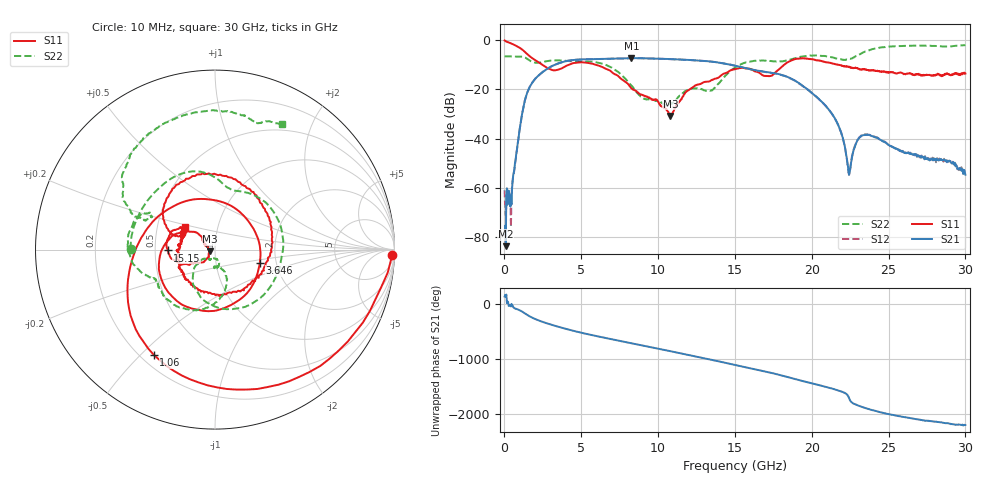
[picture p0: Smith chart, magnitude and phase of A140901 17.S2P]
!  2-Port S-parameters saved by WinCal
! VAR MeasName=S-Parameters (CALIBRATED_DATA) read from VNA (N5244A)
! VAR MeasDate=11/3/2014 9:28:11 AM
! VAR NAME=A140901 17
! VAR FILENAME=A140901 17.S2P
! VAR DATE=11/3/2014 9:28:11 AM
! VAR PHYS_PORTS=1,2
# Hz S RI R 50
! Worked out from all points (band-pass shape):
!   801 points, 10 MHz to 30 GHz, reference 50 ohm
!   highest |S21| = -7.29 dB at 8.257 GHz (marker M1); lowest = -83.7 dB at 84.97 MHz (marker M2)
!   |S21| within 3 dB of the highest: 3.168 GHz to 14.96 GHz (11.79 GHz wide, 130 % of centre)
!   lowest |S11| = -30.8 dB at 10.81 GHz (marker M3), VSWR 1.06, Z = 47.3 - j0.843 ohm
!   |S11| at or under -10 dB: 2.468 GHz to 4.195 GHz (1.727 GHz wide, 51.8 % of centre); 5.941 GHz to 18.2 GHz (12.26 GHz wide, 102 % of centre); 21.76 GHz to end of sweep
!   |S22| runs from -26.7 to -2.0 dB; largest |S21 - S12| = 0.005
!   S11 on the Smith chart (normalised r, x): 10 MHz: 21, -54; 1.06 GHz: 0.25, -0.55; 3.646 GHz: 1.64, -0.26; 15.15 GHz: 0.58, -0.01; 30 GHz: 0.69, +0.18
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1e7  0.987 -0.0321  -9.33e-05 6.74e-05  0.000723 0.00052  -0.4706 0.00357
8.4975e7  0.9268 -0.2078  -5e-05 4.15e-05  -0.000124 0.000242  -0.469 0.0396
4.5985e8  0.4703 -0.7085  0.000453 7.88e-05  0.000668 -3.1e-05  -0.4194 0.2046
1.05965e9  -0.3415 -0.5862  -0.00954 -0.0193  -0.00937 -0.0194  -0.2336 0.4021
1.546988e9  -0.4799 -0.1376  -0.0887 0.0379  -0.0887 0.0379  -0.00344 0.405
2.4092e9  -0.1957 0.2585  0.1443 0.1607  0.1438 0.1609  0.1442 0.3242
3.646288e9  0.2497 -0.0738  0.1775 -0.3009  0.1781 -0.3004  0.3702 0.113
5.033325e9  -0.2125 -0.2861  -0.3802 -0.1446  -0.3807 -0.1436  0.3164 -0.1946
6.75775e9  -0.2391 0.0767  -0.0509 0.4165  -0.0508 0.4163  -0.0446 -0.2953
8.25725e9  -0.0756 0.0734  0.4239 0.0823  0.4223 0.0827  -0.0931 -0.0756
1.001916e10  -0.0516 0.0212  0.00428 -0.4212  0.00414 -0.4204  -0.0265 -0.0522
1.08064e10  -0.0274 -0.0089  -0.2884 -0.2947  -0.288 -0.2939  0.0038 -0.0506
1.298068e10  -0.1184 -0.0747  -0.06 0.3739  -0.0601 0.3743  -0.00497 -0.0955
1.5005e10  -0.2564 -0.0245  0.2749 -0.1288  0.2714 -0.1314  0.0247 -0.277
1.515495e10  -0.2642 -0.00479  0.2448 -0.1669  0.2416 -0.1682  0.000599 -0.2954
1.732922e10  -0.1715 0.0732  -0.2134 -0.0462  -0.2117 -0.0463  -0.3151 -0.2107
2.002832e10  0.0925 0.401  0.0834 -0.00354  0.0835 -0.00272  -0.4847 0.0358
2.16028e10  0.3177 0.0459  -0.011 -0.0196  -0.0108 -0.0198  -0.3698 0.2031
2.242752e10  0.2441 -0.157  2.13e-06 0.00183  2.76e-05 0.00187  -0.377 0.168
2.325225e10  0.0622 -0.2497  0.00374 -0.0108  0.00387 -0.0108  -0.484 0.2418
2.501416e10  -0.1835 -0.1164  -0.00673 0.00297  -0.00694 0.00307  -0.3857 0.6319
3e10  -0.1672 0.1267  0.00135 -0.00126  0.00155 -0.00151  0.3737 0.6995
